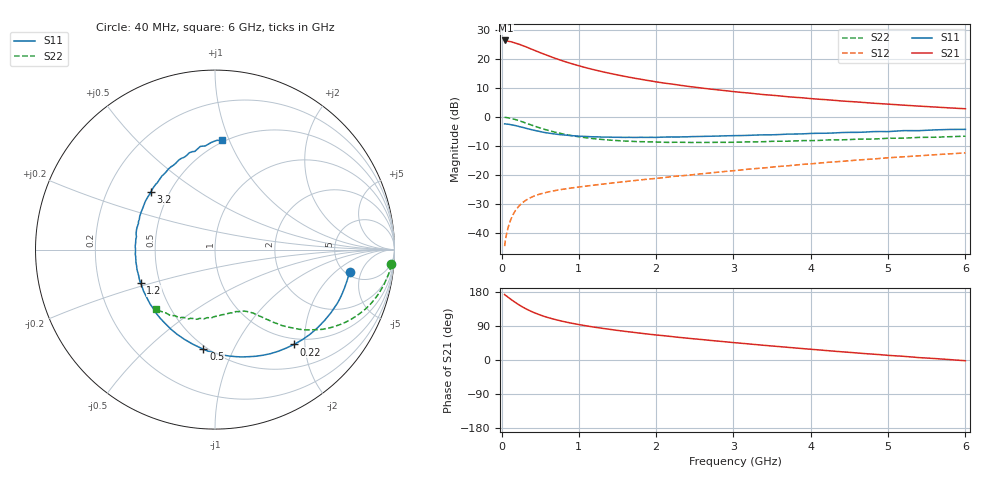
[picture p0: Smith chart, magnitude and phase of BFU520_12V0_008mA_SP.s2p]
! Filename:  P:\Prog\Test\Noise\ATS_data\Testdata_Net\03 Spar\BFU520_APG2013_37_A05_12p0V_008mA_SP_CM01_D.s2p
! Date/Time: Fri 26/Apr/2013 13:00:11
! BFU520_APG2013_37_A05_12p0V_1to20mA_SP_CM01_Bias5_R.s2p
! MDIF S-parameter v. bias file
! BFU520_APG2013_37_A05_12p0V_1to20mA_SP_CM01
! Date/time Tue Apr 23 18:22:57 2013
! VAR V_out= 12.0000
! VAR I_out= 8.0000
! VAR V_in= 0.8119
! VAR I_in= 0.0790
! Device data file deembeded for feedlines and parallel
! Original file: \03 Spar\BFU520_APG2013_37_A05_12p0V_008mA_SP_CM01_R.s2p
! Feed-files: PR047V01_250413_Feed1.s2p, PR047V01_250413_Feed2.s2p
! Parallel-file: PR047V01_250413_Par.s2p
# MHz S MA R 50
!  Freq-MHz  S11-mag  S11-arg  S21-mag  S21-arg  S12-mag  S12-arg  S22-mag  S22-arg
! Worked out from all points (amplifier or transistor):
!   98 points, 40 MHz to 6 GHz, reference 50 ohm
!   highest |S21| = 26.4 dB at 50 MHz (marker M1)
!   |S21| within 3 dB of that: start of sweep to 388.6 MHz
!   unconditionally stable (mu >= 1): 1.988 GHz to 4.13 GHz
!   at 300 MHz: K = 0.26, MSG = 26.7 dB, |S12| = -29.0 dB
!   at 1.6 GHz: K = 0.92, MSG = 18.1 dB, |S12| = -22.3 dB
!   at 6 GHz: K = 0.86, MSG = 7.6 dB, |S12| = -12.4 dB
!   S11 on the Smith chart (normalised r, x): 40 MHz: 5.39, -3.22; 220 MHz: 0.89, -1.78; 500 MHz: 0.48, -0.77; 1.2 GHz: 0.39, -0.18; 3.2 GHz: 0.39, +0.33; 6 GHz: 0.49, +0.94
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40  0.761 -9.5  20.8 172.8  0.005912 82.6  0.9829 -4.8
50  0.7573 -12.0  20.83 170.6  0.007405 81.6  0.9826 -6.1
60  0.7548 -14.1  20.46 169.5  0.008861 80.7  0.9782 -7.7
70  0.7525 -16.6  20.4 168.2  0.01021 79.8  0.9724 -8.9
140  0.7271 -33.0  19.5 157.3  0.01954 72.9  0.9312 -17.3
220  0.6877 -50.2  18.09 146.3  0.02846 65.7  0.8665 -25.5
260  0.6669 -58.1  17.26 141.4  0.0322 62.5  0.8319 -29.1
320  0.6356 -69.3  16.11 134.6  0.03694 58.6  0.78 -33.8
400  0.5982 -82.4  14.55 126.9  0.04197 54.5  0.7142 -38.6
500  0.5592 -96.6  12.84 118.9  0.04697 50.7  0.6454 -43.5
600  0.528 -108.9  11.42 112.1  0.05075 48.4  0.5885 -47.0
750  0.4965 -124.0  9.665 104.0  0.05544 46.3  0.5249 -50.9
900  0.4753 -136.4  8.34 97.3  0.05943 45.5  0.4787 -53.8
1050  0.4624 -146.9  7.314 91.7  0.06312 45.3  0.4454 -56.2
1200  0.4543 -155.8  6.496 86.7  0.06679 45.4  0.4212 -58.3
1600  0.4436 -175.0  4.983 75.5  0.07678 46.5  0.3841 -63.6
2050  0.4472 169.3  3.929 65.1  0.08849 48.0  0.3673 -70.0
3100  0.4774 139.5  2.652 44.2  0.1218 49.0  0.3689 -86.3
3200  0.4814 137.8  2.582 42.4  0.126 48.9  0.3712 -87.6
4100  0.5227 117.8  2.022 26.7  0.1595 46.2  0.3931 -102.8
5200  0.5808 98.1  1.597 9.7  0.2056 40.3  0.4302 -121.2
6000  0.6106 86.2  1.384 -1.9  0.2398 34.5  0.4657 -134.4
